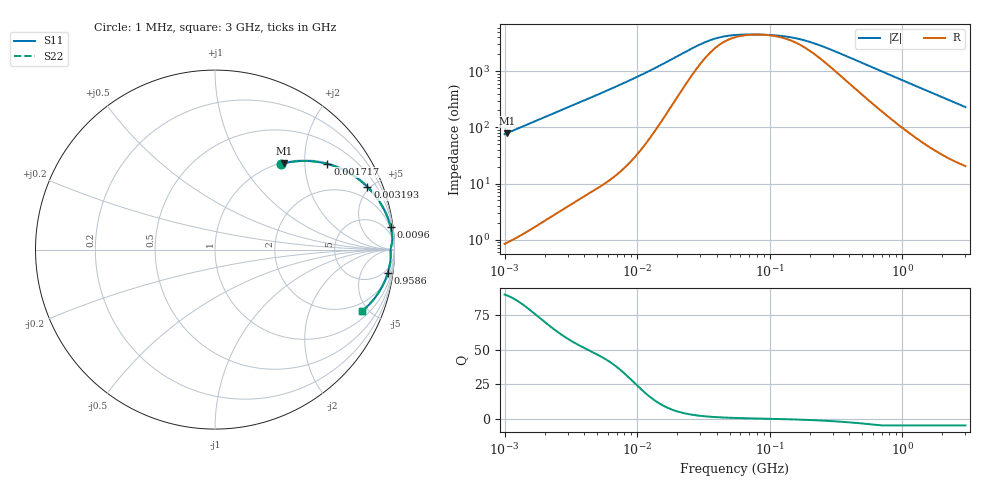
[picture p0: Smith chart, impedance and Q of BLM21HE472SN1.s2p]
! BLM21HE472SN1
# Hz S RI R 50
!Freq.(Hz) S11(Real) S11(Imag) S21(Real) S21(Imag) S12(Real) S12(Imag) S22(Real) S22(Imag)
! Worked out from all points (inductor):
!   401 points, 1 MHz to 3 GHz, reference 50 ohm
!   read as one part in series: L = 12.1 uH near 1.041 MHz
!   highest Q = 89.6 at 1.041 MHz (marker M1), where L = 12.1 uH
!   self-resonance near 84.2 MHz
!   S11 on the Smith chart (normalised r, x): 1 MHz: 1.02, +1.52; 1.717 MHz: 1.03, +2.60; 3.193 MHz: 1.09, +4.83; 9.6 MHz: 2, +15; 958.6 MHz: 3, -14; 3 GHz: 1.41, -4.59
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1000000  0.3663 0.4763  0.6337 -0.4763  0.6337 -0.4763  0.3663 0.4763
1040844  0.3849 0.481  0.6151 -0.481  0.6151 -0.481  0.3849 0.481
1323425  0.5014 0.4941  0.4986 -0.4941  0.4986 -0.4941  0.5014 0.4941
1716745  0.6268 0.4771  0.3732 -0.4771  0.3732 -0.4771  0.6268 0.4771
2364779  0.7588 0.4202  0.2412 -0.4202  0.2412 -0.4202  0.7588 0.4202
3192880  0.8495 0.3488  0.1505 -0.3488  0.1505 -0.3488  0.8495 0.3488
3823119  0.889 0.3048  0.111 -0.3048  0.111 -0.3048  0.889 0.3048
5820586  0.9474 0.2119  0.0526 -0.2119  0.0526 -0.2119  0.9474 0.2119
9600343  0.9781 0.1281  0.0219 -0.1281  0.0219 -0.1281  0.9781 0.1281
1.461624e7  0.9866 0.0788  0.0134 -0.0788  0.0134 -0.0788  0.9866 0.0788
3.320783e7  0.9836 0.0243  0.0164 -0.0243  0.0164 -0.0243  0.9836 0.0243
4.22235e7  0.9815 0.0158  0.0185 -0.0158  0.0185 -0.0158  0.9815 0.0158
5.477226e7  0.9797 0.00891  0.0203 -0.00891  0.0203 -0.00891  0.9797 0.00891
7.852918e7  0.9784 0.00135  0.0216 -0.00135  0.0216 -0.00135  0.9784 0.00135
1.171891e8  0.9782 -0.00663  0.0218 0.00663  0.0218 0.00663  0.9782 -0.00663
1.582265e8  0.9787 -0.0137  0.0213 0.0137  0.0213 0.0137  0.9787 -0.0137
2.094008e8  0.9792 -0.0221  0.0208 0.0221  0.0208 0.0221  0.9792 -0.0221
3.062963e8  0.9792 -0.0371  0.0208 0.0371  0.0208 0.0371  0.9792 -0.0371
8.005644e8  0.9687 -0.1076  0.0313 0.1076  0.0313 0.1076  0.9687 -0.1076
9.585869e8  0.9628 -0.1288  0.0372 0.1288  0.0372 0.1288  0.9628 -0.1288
1.782824e9  0.9179 -0.2296  0.0821 0.2296  0.0821 0.2296  0.9179 -0.2296
3e9  0.8208 -0.3415  0.1792 0.3415  0.1792 0.3415  0.8208 -0.3415
